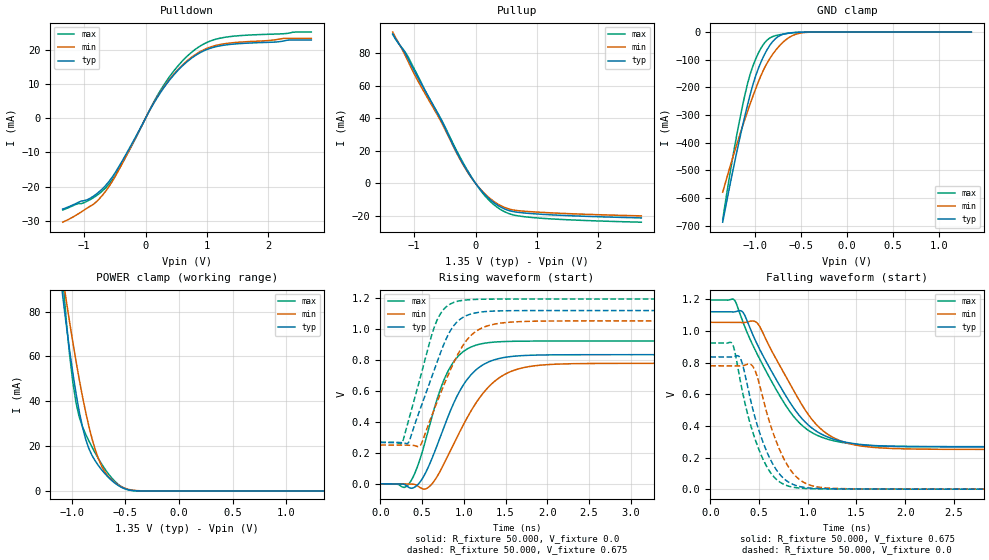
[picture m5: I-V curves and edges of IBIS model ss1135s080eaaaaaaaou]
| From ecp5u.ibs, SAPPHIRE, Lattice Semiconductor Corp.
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|   Model ss1135s080eaaaaaaaou
[Model] ss1135s080eaaaaaaaou
Model_type  Output
Polarity   Non-Inverting
Enable   Active-Low
Vmeas =  0.675V
Cref =  30.000pF
Rref =  50.000
Vref =  0.675V
C_comp   5.000pF   4.000pF   5.500pF
[Temperature Range]   25.000   0.125k   -40.000
[Voltage Range]   1.350V   1.280V   1.420V
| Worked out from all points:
|   slope of the pulldown table from 0 to 0.203 V, typ, clamps not added: 31.9 ohm
|   slope of the pullup table from 0 to 0.203 V, typ, clamps not added: 23.1 ohm
|   GND clamp passes 1 mA (typ) near -0.54 V on its own axis
|   POWER clamp passes 1 mA (typ) near -0.51 V on its own axis
|   rising waveform, R_fixture 50.000, V_fixture 0.0: 20-80 % time 409ps typ, 504ps min, 331ps max; typ from 0 V to 0.836 V
|   rising waveform, R_fixture 50.000, V_fixture 0.675: 20-80 % time 352ps typ, 392ps min, 284ps max; typ from 0.268 V to 1.12 V
|   falling waveform, R_fixture 50.000, V_fixture 0.675: 20-80 % time 496ps typ, 470ps min, 499ps max; typ from 1.12 V to 0.268 V
|   falling waveform, R_fixture 50.000, V_fixture 0.0: 20-80 % time 259ps typ, 267ps min, 253ps max; typ from 0.836 V to 0 V
[Pulldown]
|Voltage   I(typ)   I(min)   I(max)
-1.35V    -26.53mA   -30.36mA   -26.81mA
-850mV    -22.78mA   -25.14mA   -23.23mA
-600mV    -18.58mA   -20.07mA   -19.34mA
-350mV    -11.53mA   -12.21mA   -12.18mA
50mV      1.697mA    1.729mA    1.836mA
200mV     6.283mA    6.399mA    6.82mA
450mV     12.4mA     12.61mA    13.53mA
750mV     17.5mA     17.78mA    19.22mA
1V        20.02mA    20.36mA    22.09mA
1.3V      21.34mA    21.73mA    23.6mA
2.25V     22.49mA    23.26mA    24.62mA
2.7V      22.81mA    23.26mA    25.1mA
[Pullup]
|Voltage   I(typ)   I(min)   I(max)
-1.35V    91.73mA    92.83mA    91.35mA
-1.1V     76.51mA    74.91mA    77.69mA
-800mV    55.41mA    53.55mA    55.34mA
-600mV    41.59mA    40.46mA    42.07mA
-200mV    11.7mA     11.18mA    12.44mA
-100mV    5.497mA    5.179mA    5.956mA
50mV      -2.469mA   -2.291mA   -2.729mA
150mV     -6.809mA   -6.345mA   -7.521mA
300mV     -11.88mA   -11.13mA   -13.13mA
550mV     -16.74mA   -15.78mA   -18.64mA
800mV     -18.19mA   -17.11mA   -20.48mA
2.7V      -21.19mA   -19.93mA   -23.82mA
[GND_clamp]
|Voltage   I(typ)   I(min)   I(max)
-1.35V    -687.3mA   -578.9mA   -678.1mA
-1.26V    -534.3mA   -475.1mA   -489.7mA
-1.2V     -438.1mA   -409.1mA   -376.7mA
-1.08V    -262.9mA   -286.2mA   -185.9mA
-1.02V    -187.7mA   -229.9mA   -120.7mA
-960mV    -129.1mA   -177.6mA   -73.95mA
-900mV    -83.6mA    -132.1mA   -40.76mA
-840mV    -48.57mA   -96.56mA   -21.66mA
-750mV    -16.65mA   -55.68mA   -10.64mA
-660mV    -4.958mA   -26.68mA   -5.448mA
-480mV    -317.7uA   -2.229mA   -341.9uA
1.35V     0A         0A         0A
[POWER_clamp]
|Voltage   I(typ)   I(min)   I(max)
-1.35V    211.5mA    193mA      324.9mA
-1.08V    85.33mA    94.25mA    92.93mA
-1.05V    73.76mA    84.65mA    75.65mA
-990mV    52.73mA    66.45mA    48.6mA
-960mV    43.53mA    57.9mA     39.38mA
-930mV    35.42mA    49.79mA    33mA
-840mV    18.88mA    28.82mA    22.31mA
-750mV    11.24mA    14.22mA    14.3mA
-660mV    6.13mA     6.499mA    7.742mA
-570mV    2.538mA    2.795mA    3.049mA
-390mV    57.41uA    134.8uA    35.81uA
1.35V     0A         0A         0A
[Ramp]
| variable   typ   min   max
dV/dt_r   0.494/0.414n   0.460/0.507n   0.518/0.332n
dV/dt_f   0.454/0.511n   0.438/0.461n   0.496/0.548n
R_load = 50.000
[Rising Waveform]
R_fixture= 50.000
V_fixture= 0.0
V_fixture_min= 0.0
V_fixture_max= 0.0
|time   V(typ)   V(min)   V(max)
0s        0V         0V         0V
342ps     -23.61mV   -1.132mV   -951.5uV
460ps     697.3uV    -19.02mV   134.2mV
587ps     122.7mV    -18.26mV   371.1mV
728ps     317mV      93.15mV    624.6mV
867ps     507.5mV    244.5mV    780.7mV
1.238ns   772.8mV    591.3mV    908.9mV
1.587ns   824.9mV    731.8mV    922.3mV
2.127ns   834.9mV    774.7mV    923.9mV
10ns      835.7mV    779.7mV    924mV
[Rising Waveform]
R_fixture= 50.000
V_fixture= 0.675
V_fixture_min= 0.642
V_fixture_max= 0.710
|time   V(typ)   V(min)   V(max)
0s        268.3mV    251mV      268.1mV
259ps     266.8mV    250.9mV    264.2mV
339ps     268.1mV    249.9mV    411.6mV
481ps     488.7mV    250.5mV    691mV
700ps     817.5mV    556.9mV    1.082V
833ps     985.1mV    729.1mV    1.162V
960ps     1.067V     868.9mV    1.185V
1.216ns   1.112V     1.008V     1.194V
1.696ns   1.121V     1.05V      1.196V
10ns      1.121V     1.054V     1.196V
[Falling Waveform]
R_fixture= 50.000
V_fixture= 0.675
V_fixture_min= 0.642
V_fixture_max= 0.710
|time   V(typ)   V(min)   V(max)
0s        1.121V     1.054V     1.196V
251ps     1.121V     1.054V     1.193V
337ps     1.116V     1.052V     1.054V
480ps     917.3mV    1.051V     855.1mV
732ps     633.8mV    759.8mV    570.4mV
913ps     465.7mV    561.4mV    419.7mV
1.126ns   352.5mV    385.5mV    332.4mV
1.39ns    296.6mV    293.9mV    291.4mV
2.283ns   268.7mV    252.3mV    268.3mV
10ns      268.3mV    251mV      268.1mV
[Falling Waveform]
R_fixture= 50.000
V_fixture= 0.0
V_fixture_min= 0.0
V_fixture_max= 0.0
|time   V(typ)   V(min)   V(max)
0s        835.7mV    779.7mV    924mV
232ps     834.9mV    779.7mV    911.2mV
317ps     815.6mV    778.4mV    656.3mV
433ps     513.3mV    778.8mV    366.1mV
630ps     171.6mV    381.5mV    94.91mV
753ps     67.93mV    194.4mV    31.09mV
870ps     24.94mV    86.18mV    10.21mV
1.05ns    5.702mV    20.53mV    2.658mV
1.4ns     1.505mV    2.797mV    1.152mV
10ns      0V         0V         0V
